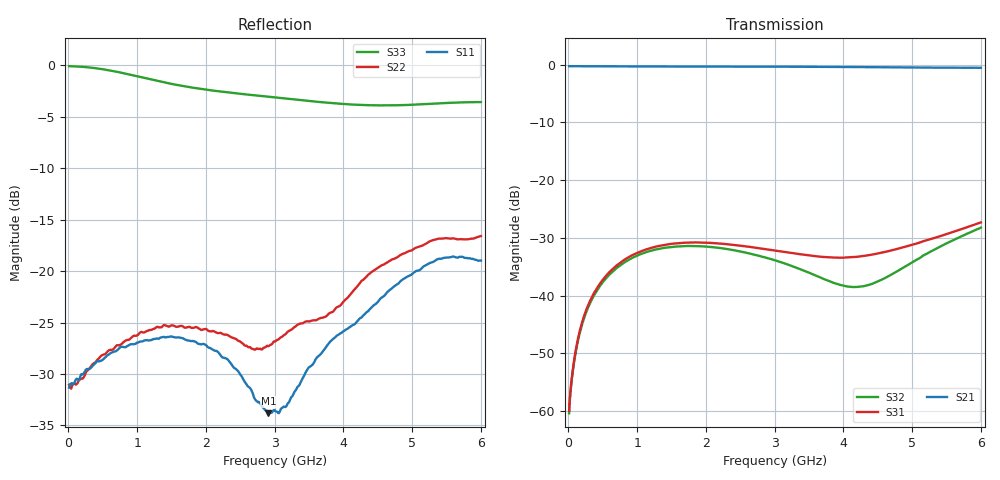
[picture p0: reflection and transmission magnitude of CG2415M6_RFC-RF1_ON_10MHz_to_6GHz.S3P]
!CEL
!CG2415M6
!Port1: RFC Port2: RF1  Port3: RF2
!Freq	S11 S12	S13 S21 S22 S23 S31 S32 S33
# Hz S dB R 50
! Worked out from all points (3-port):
!   600 points, 10 MHz to 6 GHz, reference 50 ohm
!   strongest paths, dB at 10 MHz, 1.51 GHz, 3.01 GHz, 4.51 GHz, 6 GHz:
!     S21: -0.3, -0.3, -0.4, -0.4, -0.5
!     S31: -60.0, -31.0, -32.2, -32.7, -27.3
!     S32: -60.4, -31.5, -33.9, -37.5, -28.2
!   lowest |S11| = -33.8 dB at 2.91 GHz (marker M1), VSWR 1.04, Z = 51 + j1.78 ohm
!   |S11| at or under -10 dB: start of sweep to end of sweep
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1e7  -31.32 1.3  -0.27 -0.2  -59.98 20.7
     -0.27 -0.2  -31.05 -1.3  -60.35 20.1
     -59.97 19.8  -60.36 20.5  -0.07 -0.8
1.1e8  -30.52 12.9  -0.28 -1.1  -49.17 64.7
       -0.28 -1.1  -31.03 12.1  -49.54 64.4
       -49.17 64.9  -49.53 64.6  -0.10 -7.6
2.5e8  -29.63 23.7  -0.29 -2.3  -42.74 70.4
       -0.29 -2.3  -29.91 26.1  -43.14 69.4
       -42.74 70.5  -43.14 69.7  -0.16 -17.2
7.6e8  -27.37 44.3  -0.31 -6.7  -34.22 58.8
       -0.31 -6.7  -27.14 42.0  -34.65 56.5
       -34.23 58.8  -34.70 56.6  -0.69 -51.4
1.21e9  -26.69 45.6  -0.33 -10.4  -31.71 46.6
        -0.33 -10.4  -25.70 41.6  -32.19 43.2
        -31.70 46.6  -32.19 43.1  -1.38 -79.6
1.78e9  -26.80 48.7  -0.34 -15.1  -30.80 36.2
        -0.34 -15.1  -25.49 35.2  -31.42 30.4
        -30.80 36.1  -31.40 30.2  -2.13 -109.3
2.91e9  -33.83 58.9  -0.36 -24.6  -31.98 31.4
        -0.36 -24.7  -27.30 4.2  -33.48 19.5
        -32.01 31.2  -33.55 19.4  -3.05 -149.6
3.01e9  -33.61 60.1  -0.37 -25.5  -32.17 32.2
        -0.36 -25.5  -26.83 2.2  -33.84 19.7
        -32.19 31.9  -33.90 19.6  -3.11 -152.6
4.27e9  -24.46 77.4  -0.44 -36.5  -33.16 58.7
        -0.43 -36.6  -20.92 7.4  -38.46 64.2
        -33.16 58.5  -38.41 64.4  -3.84 168.5
6e9  -18.97 59.3  -0.54 -52.0  -27.34 82.1
     -0.55 -52.1  -16.59 -1.6  -28.23 107.5
     -27.32 81.6  -28.22 106.4  -3.56 128.9
